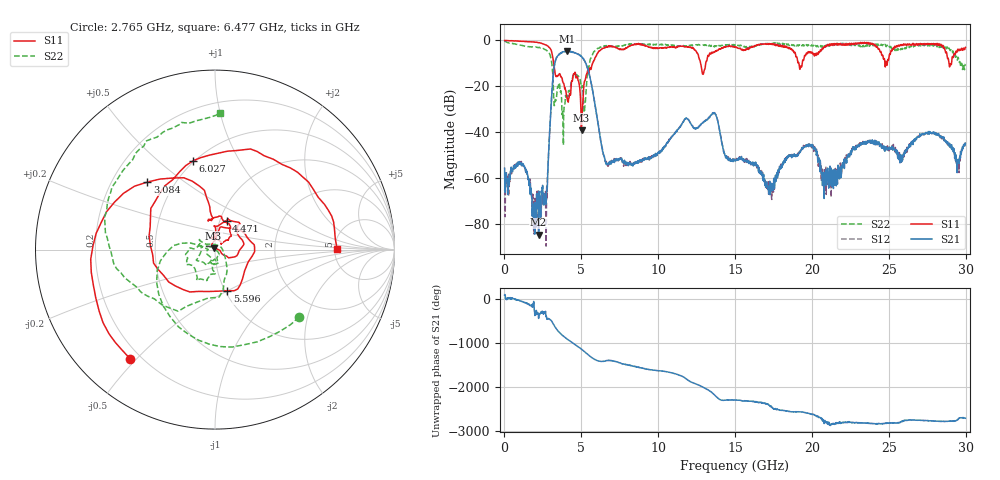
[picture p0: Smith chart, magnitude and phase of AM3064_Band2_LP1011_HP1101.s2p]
# Hz S DB R 50.0
!freq dBS11 angS11 dBS21 angS21 dBS12 angS12 dBS22 angS22
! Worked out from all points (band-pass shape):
!   1600 points, 10 MHz to 29.98 GHz, reference 50 ohm
!   highest |S21| = -4.72 dB at 4.077 GHz (marker M1); lowest = -84.6 dB at 2.222 GHz (marker M2)
!   |S21| within 3 dB of the highest: 3.376 GHz to 5.102 GHz (1.726 GHz wide, 40.7 % of centre)
!   lowest |S11| = -39.2 dB at 5.015 GHz (marker M3), VSWR 1.02, Z = 49.2 + j0.757 ohm
!   |S11| at or under -10 dB: 3.206 GHz to 5.732 GHz (2.526 GHz wide, 56.5 % of centre); 12.76 GHz to 13.09 GHz (330 MHz wide, 2.55 % of centre); 19.15 GHz to 19.37 GHz (217.5 MHz wide, 1.13 % of centre)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
!   |S22| runs from -45.6 to -0.3 dB; largest |S21 - S12| = 0.014
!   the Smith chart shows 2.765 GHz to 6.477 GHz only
!   S11 on the Smith chart (normalised r, x): 2.765 GHz: 0.16, -0.48; 3.084 GHz: 0.35, +0.37; 4.471 GHz: 1.08, +0.36; 5.596 GHz: 1.02, -0.50; 6.027 GHz: 0.49, +0.66; 6.477 GHz: 5.26, +0.05
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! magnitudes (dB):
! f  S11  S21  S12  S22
! 10 MHz  0.0  -55.6  -65.0  -0.3
! 1.078 GHz  -0.4  -53.3  -54.0  -2.2
! 2.222 GHz  -1.0  -84.6  -67.3  -3.1
! 2.765 GHz  -2.3  -64.4  -68.6  -4.4
! 3.084 GHz  -5.5  -22.7  -22.5  -10.2
! 3.384 GHz  -15.5  -7.5  -7.5  -25.0
! 4.077 GHz  -25.2  -4.7  -4.8  -24.6
! 4.471 GHz  -15.2  -5.2  -5.1  -15.1
! 5.015 GHz  -39.2  -7.2  -7.0  -20.8
! 5.596 GHz  -12.4  -17.1  -17.0  -8.0
! 6.027 GHz  -5.9  -33.7  -33.6  -3.6
! 6.477 GHz  -3.3  -50.6  -50.4  -2.4
! 10 GHz  -3.4  -49.1  -49.4  -1.9
! 12.92 GHz  -14.8  -35.8  -35.7  -2.0
! 13.6 GHz  -5.1  -31.9  -31.6  -2.6
! 15 GHz  -2.7  -52.5  -52.7  -1.9
! 17.33 GHz  -1.6  -65.1  -65.4  -1.5
! 19.99 GHz  -5.1  -45.9  -46.1  -1.9
! 20.98 GHz  -2.3  -58.2  -58.7  -2.7
! 23.03 GHz  -1.3  -45.3  -45.3  -2.5
! 25 GHz  -8.1  -47.0  -47.1  -2.3
! 29.98 GHz  -3.0  -44.8  -46.0  -10.3
